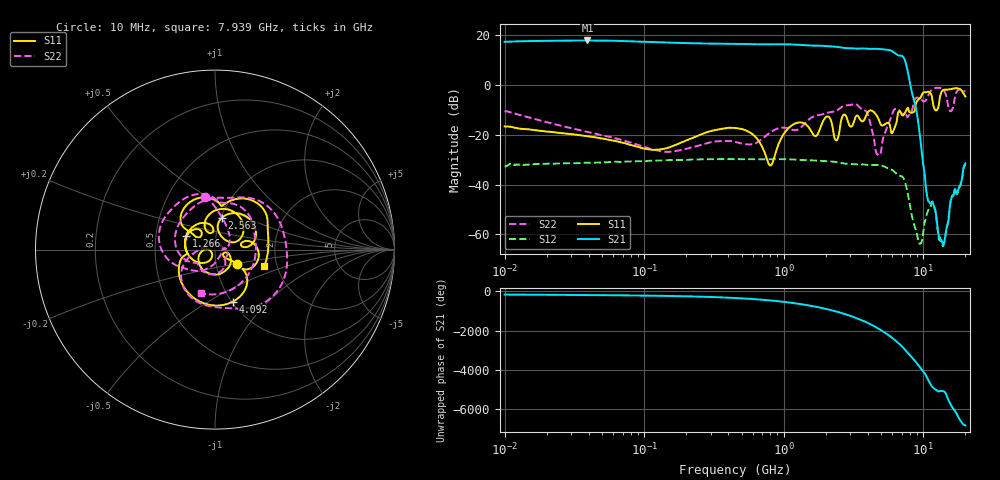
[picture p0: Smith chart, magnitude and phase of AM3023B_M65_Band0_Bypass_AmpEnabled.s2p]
!Agilent Technologies,E8364B,MY43040894,A.07.50.67
!Agilent E8364B: A.07.50.67
!Date: Tuesday, October 27, 2020 10:51:45
!Correction: S11(Full 2 Port(1,2))
!S21(Full 2 Port(1,2))
!S12(Full 2 Port(1,2))
!S22(Full 2 Port(1,2))
!S2P File: Measurements: S11, S21, S12, S22:Log Frequency Sweep
# Hz S  dB  R 50
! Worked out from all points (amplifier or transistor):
!   3201 points, 10 MHz to 20 GHz, reference 50 ohm
!   highest |S21| = 18.0 dB at 39.19 MHz (marker M1)
!   |S21| within 3 dB of that: start of sweep to 2.7 GHz
!   unconditionally stable (mu >= 1): start of sweep to end of sweep
!   at 35.47 MHz: K = 2.38, MAG = 18.1 dB, |S12| = -31.3 dB
!   at 447.2 MHz: K = 2.30, MAG = 16.7 dB, |S12| = -29.7 dB
!   at 20 GHz: K = 214.43, MAG = -26.1 dB, |S12| = -31.9 dB
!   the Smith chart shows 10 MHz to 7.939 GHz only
!   S11 on the Smith chart (normalised r, x): 10 MHz: 1.26, -0.21; 1.266 GHz: 0.72, +0.11; 2.563 GHz: 1.01, +0.37; 4.092 GHz: 1.01, -0.65; 7.939 GHz: 1.71, -0.35
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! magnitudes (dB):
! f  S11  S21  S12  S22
! 10 MHz  -16.6  17.5  -32.7  -10.4
! 35.55 MHz  -20.2  18.0  -31.3  -18.2
! 39.19 MHz  -20.5  18.0  -31.1  -18.8
! 126.1 MHz  -25.9  17.3  -30.3  -26.4
! 447.2 MHz  -17.2  16.6  -29.7  -22.7
! 802.2 MHz  -32.3  16.5  -29.8  -18.9
! 1.266 GHz  -15.0  16.3  -30.0  -17.8
! 1.59 GHz  -19.0  15.9  -30.2  -12.9
! 2.07 GHz  -12.6  15.7  -30.5  -11.0
! 2.381 GHz  -22.2  15.4  -30.9  -10.3
! 2.563 GHz  -14.8  15.2  -31.2  -9.0
! 4.092 GHz  -10.3  14.6  -32.1  -13.5
! 4.753 GHz  -13.4  14.6  -32.1  -28.1
! 5.639 GHz  -15.2  14.2  -33.5  -15.3
! 7.168 GHz  -12.1  11.4  -37.2  -11.4
! 7.939 GHz  -10.7  2.2  -47.1  -11.8
! 9.464 GHz  -5.2  -20.5  -63.7  -5.3
! 10.71 GHz  -2.6  -45.4  -51.0  -4.8
! 11.75 GHz  -7.9  -47.7  -47.8  -1.5
! 13.45 GHz  -3.0  -62.3  -63.5  -1.3
! 15.66 GHz  -1.6  -46.8  -46.7  -10.5
! 20 GHz  -4.5  -31.5  -31.9  -2.6
